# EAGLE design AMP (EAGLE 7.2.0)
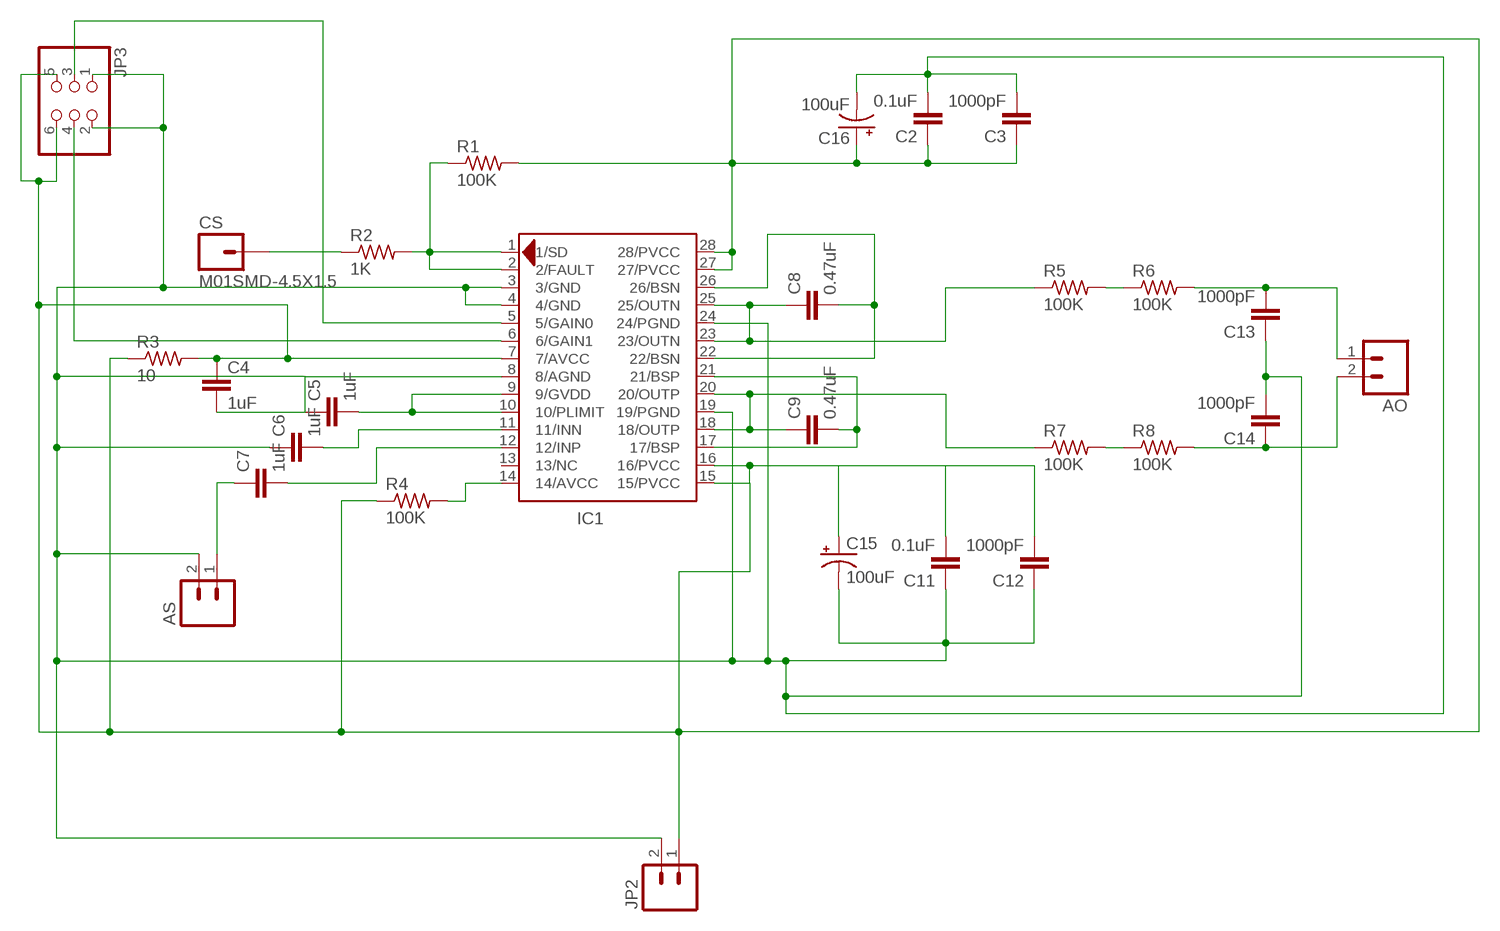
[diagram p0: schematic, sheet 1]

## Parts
AO  M02  [1X02_LONGPADS]
AS  M02  [1X02_LONGPADS]
C2  0.1uF  CAP1206  [1206]
C3  1000pF  CAP1206  [1206]
C4  1uF  CAP1206  [1206]
C5  1uF  CAP1206  [1206]
C6  1uF  CAP1206  [1206]
C7  1uF  CAP1206  [1206]
C8  0.47uF  CAP1206  [1206]
C9  0.47uF  CAP1206  [1206]
C11  0.1uF  CAP1206  [1206]
C12  1000pF  CAP1206  [1206]
C13  1000pF  CAP1206  [1206]
C14  1000pF  CAP1206  [1206]
C15  100uF  CAP_POLD  [PANASONIC_D]
C16  100uF  CAP_POLD  [PANASONIC_D]
CS  M01SMD-4.5X1.5  [PAD-1.5X4.5]
IC1  TPA3111D1  [TSSOP28-PWP]
JP2  M02  [1X02_LONGPADS]
JP3  PINHD-2X3-SMD  [2X03SMD]
R1  100K  R-US_M1206  [M1206]
R2  1K  R-US_M1206  [M1206]
R3  10  R-US_M1206  [M1206]
R4  100K  R-US_M1206  [M1206]
R5  100K  R-US_M1206  [M1206]
R6  100K  R-US_M1206  [M1206]
R7  100K  R-US_M1206  [M1206]
R8  100K  R-US_M1206  [M1206]

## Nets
GND': AS.2 C2.2 C3.2 C4.2 C5.1 C6.1 C11.1 C12.1 C13.1 C14.2 C15.- C16.- IC1.3(3/GND) IC1.4(4/GND) IC1.8(8/AGND) IC1.19(19/PGND) IC1.24(24/PGND) JP2.2 JP3.1 JP3.2
N$1: IC1.1(1/SD) IC1.2(2/FAULT) R1.1 R2.2
N$2: C5.2 IC1.9(9/GVDD) IC1.10(10/PLIMIT)
N$3: C6.2 IC1.11(11/INN)
N$4: C7.2 IC1.12(12/INP)
N$5: IC1.14(14/AVCC) R4.2
N$6: C8.1 IC1.23(23/OUTN) IC1.25(25/OUTN) R5.1
N$7: C8.2 IC1.22(22/BSN) IC1.26(26/BSN)
N$8: C9.2 IC1.17(17/BSP) IC1.21(21/BSP)
N$9: C9.1 IC1.18(18/OUTP) IC1.20(20/OUTP) R7.1
N$11: AO.2 C14.1 R8.2
N$12: R5.2 R6.1
N$13: R7.2 R8.1
N$14: IC1.5(5/GAIN0) JP3.3
N$15: IC1.6(6/GAIN1) JP3.4
N$16: CS.P$1 R2.1
N$17: AS.1 C7.1
N$18: AO.1 C13.2 R6.2
PVCC: C2.1 C3.1 C4.1 C11.2 C12.2 C15.+ C16.+ IC1.7(7/AVCC) IC1.15(15/PVCC) IC1.16(16/PVCC) IC1.27(27/PVCC) IC1.28(28/PVCC) JP2.1 JP3.5 JP3.6 R1.2 R3.1 R3.2 R4.1
Unconnected: IC1.13(13/NC)

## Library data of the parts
AO AS JP2 = 01_SparkFun:M02: Header 2
C2-C9 C11-C14 = 01_SparkFun:CAP: Capacitor
C15 C16 = 01_SparkFun:CAP_POL: Capacitor Polarized
CS = 01_SparkFun:M01: Header 1
IC1 = Audio-Power-amlifier V.2.0:TPA3111D1: 10-W FILTER-FREE MONO CLASS-D AUDIO POWER AMPLIFIER with SPEAKER GUARnd
JP3 = 01_fab:PINHD-2X3-SMD: PIN HEADER
R1-R8 = 01_adafruit:R-US_: RESISTOR, American symbol

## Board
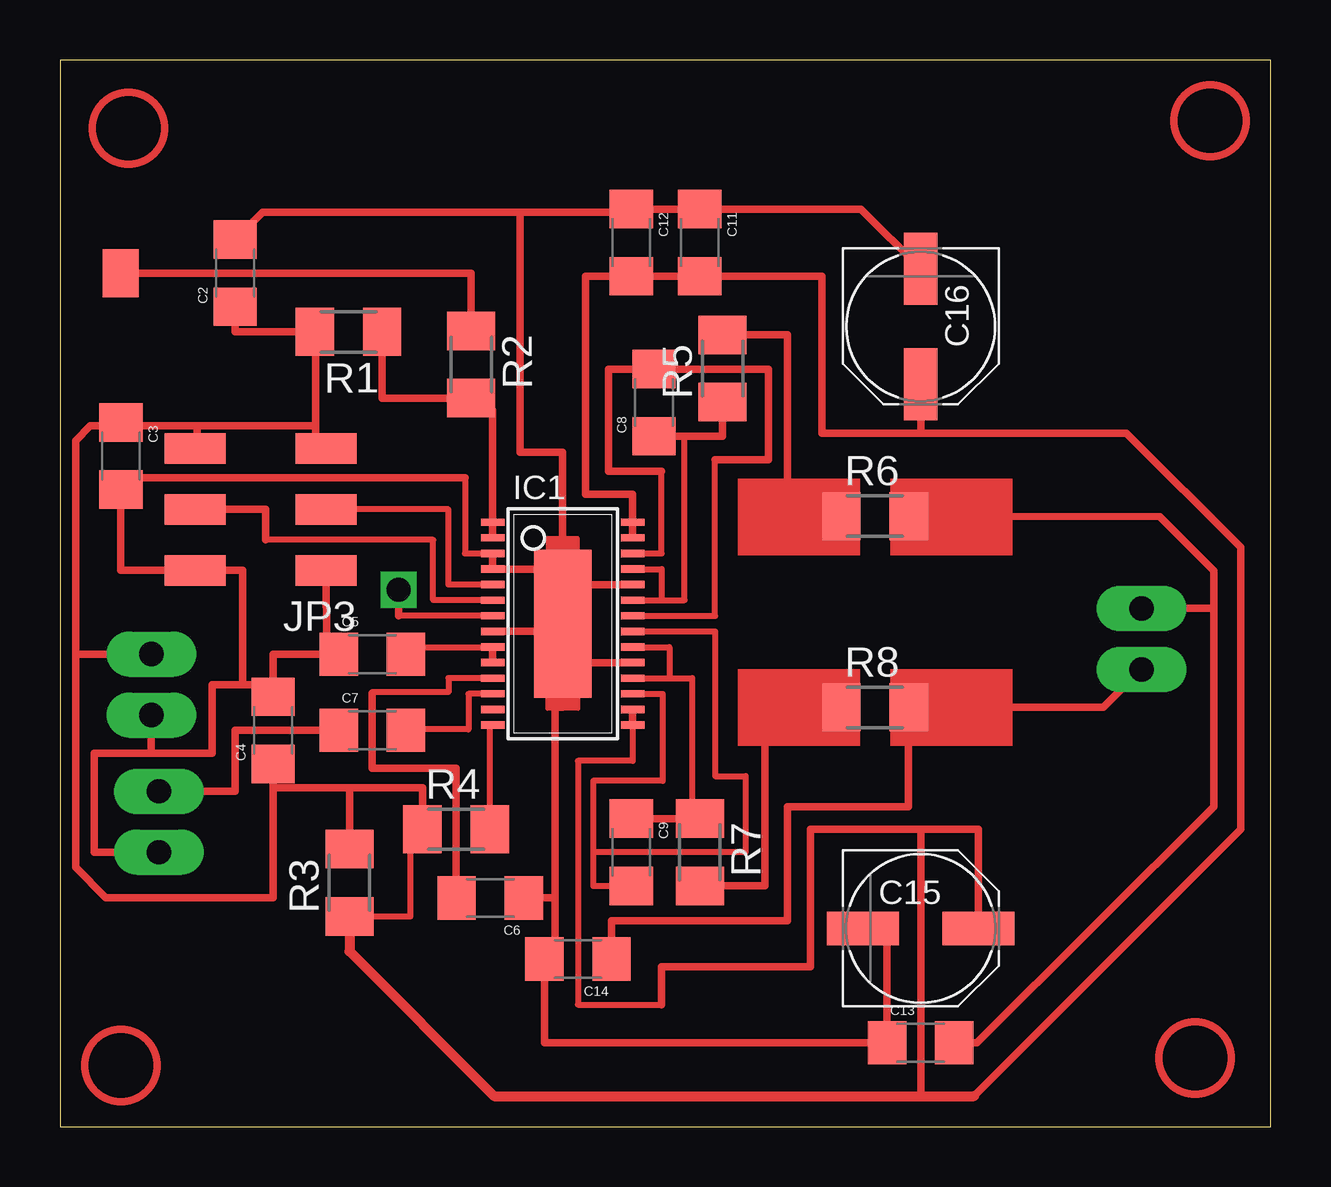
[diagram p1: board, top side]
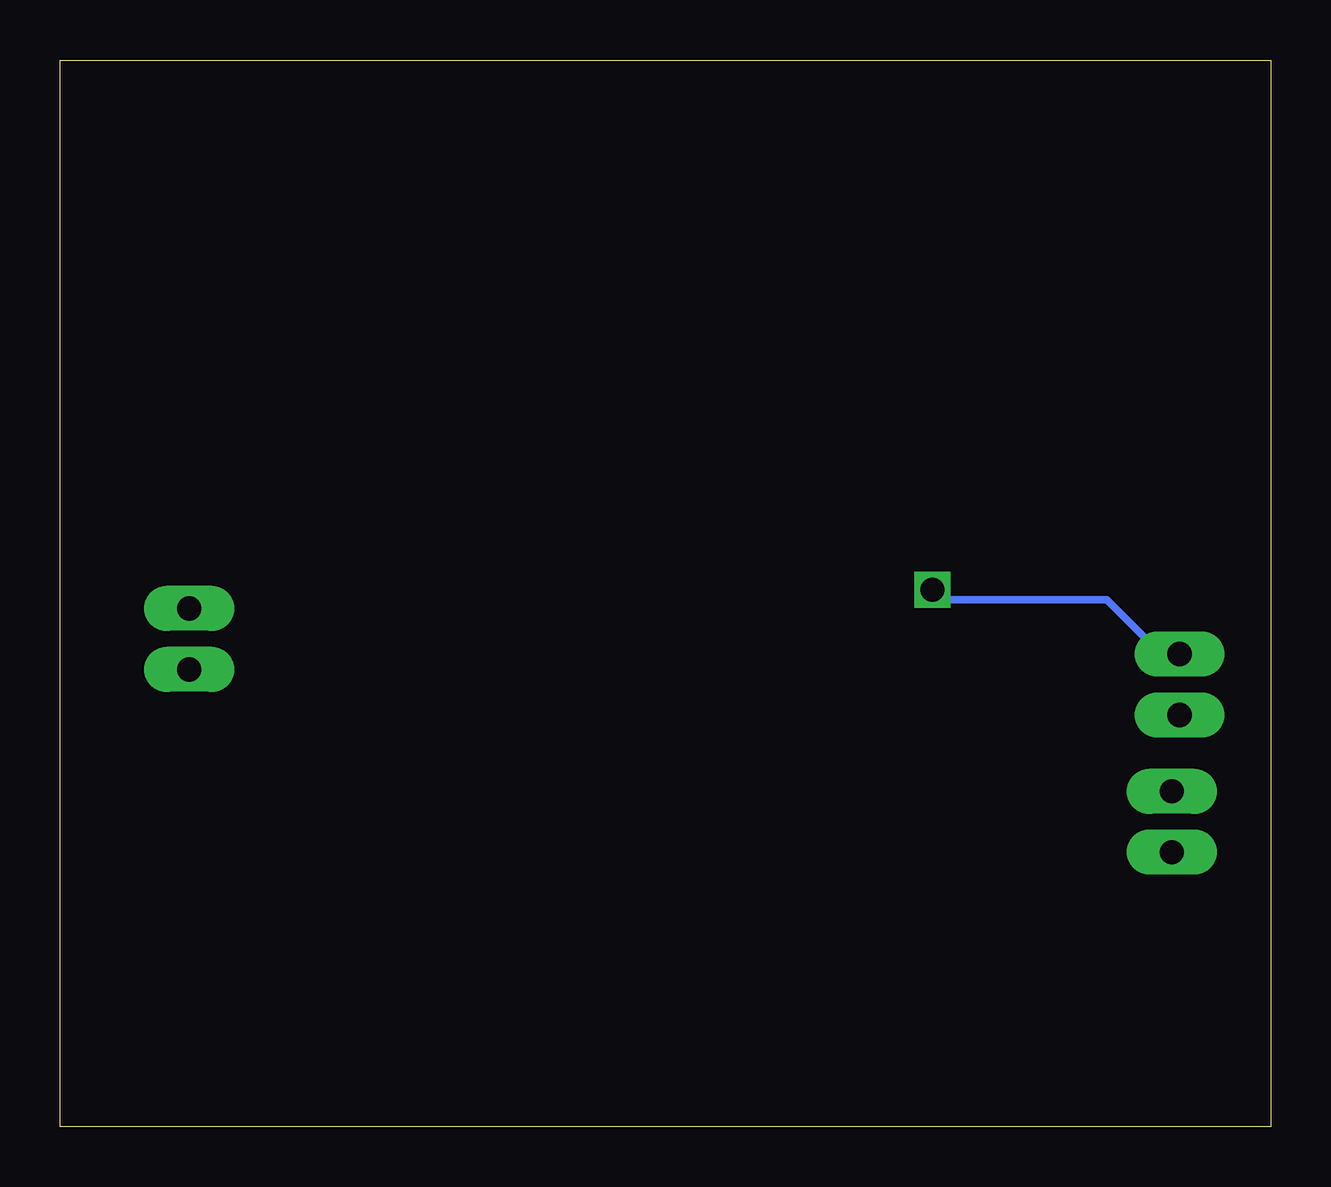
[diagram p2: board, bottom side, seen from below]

Size 50.47 x 44.44 mm. Coordinates in mm from the lower left corner, seen from the top.
Outline: 0,0 50.47,0 50.47,44.44 0,44.44 0,0
Copper layers (1*16): Top 0.035mm / dielectric 1.5mm / Bottom 0.035mm
Design rules "default *": minimum track width 12mil, minimum drill 24mil, track to track 16mil, track to pad 16mil, pad to pad 16mil, via to via 16mil, smd to smd 16mil, copper to edge 40mil, drill to drill 8mil, minimum pad ring 10mil, minimum via ring 8mil, stop-mask expansion 4mil, vias tented up to drill 0mil, thermal gap 10mil

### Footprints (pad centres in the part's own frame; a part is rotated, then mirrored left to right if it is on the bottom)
1X02_LONGPADS = drill 1.016 pad 1.88 long: 1 0,0; 2 2.54,0
1206 = smd 1.6 x 1.8: 1 -1.4,0; 2 1.4,0
PANASONIC_D = smd 3 x 1.4: + 2.4,0; - -2.4,0
PAD-1.5X4.5 = smd 1.5 x 2: P$1 0,0
TSSOP28-PWP = smd 0.305 x 0.991: 1 -4.225,-2.918; 2 -3.575,-2.918; 3 -2.925,-2.918; 4 -2.275,-2.918; 5 -1.625,-2.918; 6 -0.975,-2.918; 7 -0.325,-2.918; 8 0.325,-2.918; 9 0.975,-2.918; 10 1.625,-2.918; 11 2.275,-2.918; 12 2.925,-2.918; 13 3.575,-2.918; 14 4.225,-2.918; 15 4.225,2.918; 16 3.575,2.918; 17 2.925,2.918; 18 2.275,2.918; 19 1.625,2.918; 20 0.975,2.918; 21 0.325,2.918; 22 -0.325,2.918; 23 -0.975,2.918; 24 -1.625,2.918; 25 -2.275,2.918; 26 -2.925,2.918; 27 -3.575,2.918; 28 -4.225,2.918 | smd 6.17 x 2.4: EXP 0,0
2X03SMD = smd 2.54 x 1.27: 1 -2.54,2.54; 2 2.92,2.54; 3 -2.54,0; 4 2.92,0; 5 -2.54,-2.54; 6 2.92,-2.54
M1206 = smd 1.6 x 2: 1 -1.4,0; 2 1.4,0

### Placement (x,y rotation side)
AO  45.09,21.59 270 top
AS  4.13,13.97 270 top
C2  7.3,35.56 90 top
C3  2.54,27.94 270 top
C4  8.89,16.51 90 top
C5  13.02,19.68 0 top
C6  17.93,9.53 180 top
C7  13.02,16.51 0 top
C8  24.77,30.16 90 top
C9  23.81,11.43 270 top
C11  26.67,36.83 270 top
C12  23.81,36.83 270 top
C13  35.88,3.49 0 top
C14  21.59,6.99 180 top
C15  35.88,8.26 0 top
C16  35.88,33.34 270 top
CS  2.54,35.56 0 top
IC1  20.95,20.95 270 top
JP2  3.81,19.68 270 top
JP3  8.56,25.72 180 top
R1  12.03,33.11 180 top
R2  17.14,31.75 270 top
R3  12.06,10.16 90 top
R4  16.51,12.38 0 top
R5  27.62,31.58 90 top
R6  33.97,25.44 0 top
R7  26.67,11.43 270 top
R8  33.97,17.46 0 top

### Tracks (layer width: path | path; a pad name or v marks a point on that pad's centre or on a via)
GND'
  Top 0.254: 16.88,27.03 16.88,23.88 IC1.3
  Top 0.305: 7.62,18.41 7.62,23.18 JP3.2 2.54,23.18 C3.2 2.54,27.03 16.88,27.03 | 7.62,18.41 8.26,18.41 C4.2 8.89,19.68 C5.1 11.11,20 JP3.1 | AS.2 1.44,11.43 1.44,15.56 3.81,15.56 | 3.81,15.56 6.35,15.56 6.35,18.41 7.62,18.41 | JP2.2 3.81,15.56 | 20.95,19.33 20.95,17.46 20.64,17.46 20.64,9.53 | 20.95,19.33 IC1.19 | IC1.24 20.95,22.58 | 20.95,22.58 20.95,20.63 | 20.95,20.63 20.95,19.33 | 20.95,23.23 IC1.4 IC1.3 | 20.95,23.23 20.95,22.58 | IC1.8 20.95,20.63 | 19.18,38.1 19.18,28.11 20.95,28.11 20.95,23.23 | 19.18,38.1 23.81,38.1 C12.1 C11.1 33.38,38.23 C16.- | C15.- 34.48,8.26 C13.1 20.19,3.49 C14.2 20.64,6.99 20.64,9.53 | 19.18,38.1 8.44,38.1 C2.2 | C6.1 20.64,9.53
N$1
  Top 0.305: IC1.2 IC1.1 18.04,29.84 17.14,29.84 R2.2 13.43,30.35 R1.1
N$2
  Top 0.254: 14.73,19.33 14.73,19.98 IC1.9
  Top 0.305: 14.73,19.33 C5.2 | IC1.9 IC1.10
N$3
  Top 0.254: IC1.11 16.19,18.68 16.19,18.1 13.02,18.1 13.02,18.05
  Top 0.305: 13.02,18.05 13.02,14.92 16.51,14.92 16.51,9.86 | 16.51,9.86 16.51,9.84 | C6.2 16.43,9.86 16.51,9.86
N$4
  Top 0.254: IC1.12 17.03,18.03 17.03,16.55 14.42,16.55 C7.2
N$5
  Top 0.254: 17.91,16.73 R4.2
  Top 0.305: IC1.14 17.91,16.73
N$6
  Top 0.254: IC1.25 25.08,23.23 25.08,21.93 | IC1.23 25.08,21.93 | 25.08,21.93 26.04,21.93 26.04,28.76
  Top 0.305: C8.1 26.04,28.76 27.62,28.76 R5.1
N$7
  Top 0.254: IC1.26 25.08,23.88 25.08,27.3 | IC1.22 27.3,21.28 27.3,27.77
  Top 0.305: 27.3,27.77 29.53,27.77 29.53,31.56 C8.2 22.86,31.56 22.86,27.3 25.08,27.3
N$8
  Top 0.254: IC1.21 27.3,20.63 27.3,14.61 28.57,14.61 28.57,11.43 22.23,11.43 | IC1.17 25.12,18.03 25.12,14.4 22.23,14.4 22.23,11.43 | 22.23,11.43 22.23,10.03 C9.2
N$9
  Top 0.254: IC1.18 25.4,18.68 | 25.4,18.68 26.35,18.68 26.35,12.83 R7.1 | IC1.20 25.4,19.98 25.4,18.68
  Top 0.305: C9.1 R7.1
N$11
  Top 0.305: C14.1 22.99,8.57 30.32,8.57 30.32,13.34 35.37,13.34 R8.2 43.5,17.46 AO.2
N$12
  Top 0.305: R5.2 30.33,33 30.33,25.72 R6.1
N$13
  Top 0.305: R7.2 29.38,10.03 29.38,17.46 R8.1
N$14
  Top 0.254: IC1.5 16.19,22.58 16.19,25.72 JP3.3
N$15
  Top 0.254: IC1.6 15.56,21.93 15.56,24.45 8.57,24.45
  Top 0.305: JP3.4 8.57,25.72 8.57,24.45
N$16
  Top 0.305: CS.P$1 17.14,35.56 R2.1
N$17
  Top 0.305: C7.1 7.3,16.51 7.3,13.97 AS.1
N$18
  Top 0.305: AO.1 48.09,21.59 | 48.09,21.59 48.09,13.34 38.23,3.49 C13.2 | R6.2 45.85,25.4 48.09,23.16 48.09,21.59
PVCC  (via drill 1)
  Top 0.254: IC1.7 14.11,21.28 | IC1.16 23.87,15.24 21.59,15.24 21.59,5.08 25.08,5.08 | R3.1 14.61,8.76 14.61,12.06 15.11,12.06 R4.1
  Top 0.305: IC1.27 IC1.28 23.87,26.35 21.91,26.35 21.91,35.43 C12.2 C11.2 31.75,35.43 31.75,28.89 35.88,28.89 | IC1.16 IC1.15 | 8.26,15.24 C4.1 8.89,14.12 | 12.06,14.12 15.11,14.12 R4.1 | 2.54,29.21 1.27,29.21 0.65,28.57 0.65,19.68 | 2.54,29.21 5.71,29.21 | JP3.6 5.71,28.26 5.71,29.21 | JP3.5 10.66,28.26 10.66,29.21 | 8.89,14.12 12.06,14.12 | R3.2 12.06,14.12 | 2.54,29.21 C3.1 3.17,29.66 | 0.65,19.68 0.65,10.79 1.91,9.53 8.89,9.53 8.89,14.12 | JP2.1 0.65,19.68 | 14.11,21.28 v14.11,22.38 | 10.66,29.21 10.66,33.11 R1.2 | 5.71,29.21 10.66,29.21 | R1.2 10.63,32.89 | 38.1,1.27 49.21,12.38 49.21,24.14 44.45,28.89 35.88,28.89 | 25.08,5.08 25.08,6.67 31.28,6.67 31.28,12.38 35.88,12.38 | 35.88,1.27 35.88,12.38 | C15.+ 38.28,12.38 35.88,12.38 | C16.+ 35.88,28.89 | C2.1 7.3,33.11 R1.2
  Top 0.406: 38.1,1.27 35.88,1.27 18.1,1.27 12.06,7.3 R3.1
  Bottom 0.305: v14.11,22.38 14.3,21.95 6.83,21.95 4.7,19.81 JP2.1
(copper drawn outside any net)
  shapes: Top area x4, Top circle x4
